(* Logix 5000 Rung export; software revision 16.04 *)

TYPE MNETCDATETIME :   // Stores the date and time value
STRUCT
   Year : DINT;   // Displays module current year
   Month : DINT;   // Displays Module current month
   Day : DINT;   // Displays Module current day
   Hour : DINT;   // Displays Module current hour
   Minute : DINT;   // Displays Module current minute
   Seconds : DINT;   // Displays Module current second
END_STRUCT
END_TYPE

TYPE MNETCETHERNETTYPE :   // Allows read/write Ethernet settings between the module and processor
STRUCT
   Read : BOOL;   // Enable Ethernet configuration transfer from module to processor
   Write : BOOL;   // Enable Ethernet configuration transfer from processor to module
   Config : MNETCETHERNET;   // Module ethernet configurations ip, netmask and gateway
END_STRUCT
END_TYPE

TYPE MNETCCLOCKTYPE :   // Allows read/write of clock value between the module and processor
STRUCT
   Read : BOOL;   // Reads current time from the module
   Write : BOOL;   // Writes current time from the module
   Config : MNETCDATETIME;   // Date and time configuration read or written between the module and processor
END_STRUCT
END_TYPE

TYPE MNETCETHERNET :   // Stores the MVI56E-MNETC IP settings
STRUCT
   IP : INT[4];   // Module IP address
   Netmask : INT[4];   // Net mask used by the Module
   Gateway : INT[4];   // Gateway used by the module
END_STRUCT
END_TYPE

ADD_ON_INSTRUCTION AOI56EMNETC_Optional   (* revision 1.0, vendor ProSoft Technology Inc. *)
// MVI56E-MNETC Optional Add-On Ethernet/Clock
// Revision note:
// v1.0 - Release.
VAR_IN_OUT
   MVI56MNETCEthernet : MNETCETHERNETTYPE; {required}   // MVI56E-MNET Rev2 Ethernet Settings
   MVI56MNETCClock : MNETCCLOCKTYPE; {required}   // MVI56E-MNET Rev2 Clock Settings
   ReadEthernetMSG : MESSAGE; {required}   // Read Ethernet Settings Message
   WriteEthernetMSG : MESSAGE; {required}   // Write Ethernet Settings Message
   ReadClockMSG : MESSAGE; {required}   // Read Clock Settings Message
   WriteClockMSG : MESSAGE; {required}   // Write Clock Settings Message
END_VAR

ROUTINE Logic   (* ladder *)
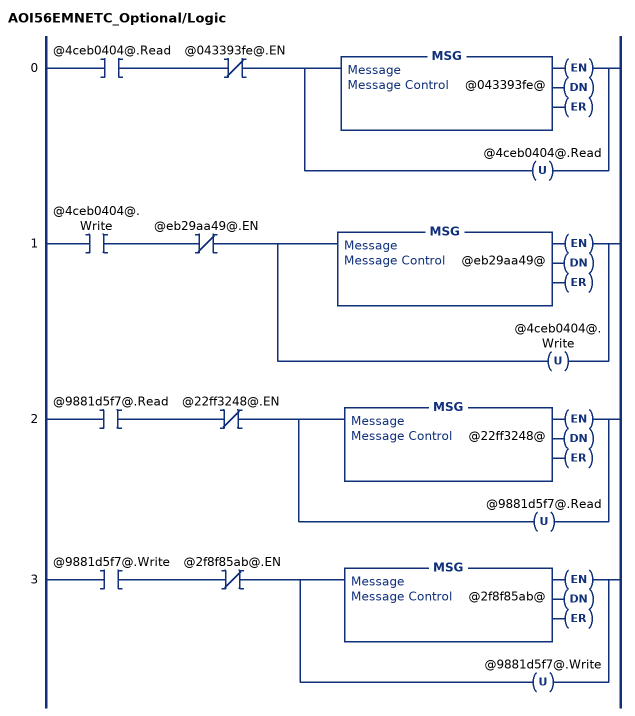
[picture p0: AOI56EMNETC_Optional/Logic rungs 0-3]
   0: XIC(@4ceb0404@.Read)XIO(@043393fe@.EN)[MSG(@043393fe@) ,OTU(@4ceb0404@.Read) ];
   1: XIC(@4ceb0404@.Write)XIO(@eb29aa49@.EN)[MSG(@eb29aa49@) ,OTU(@4ceb0404@.Write) ];
   2: XIC(@9881d5f7@.Read)XIO(@22ff3248@.EN)[MSG(@22ff3248@) ,OTU(@9881d5f7@.Read) ];
   3: XIC(@9881d5f7@.Write)XIO(@2f8f85ab@.EN)[MSG(@2f8f85ab@) ,OTU(@9881d5f7@.Write) ];
END_ROUTINE
END_ADD_ON_INSTRUCTION

VAR_GLOBAL   (* controller tags *)
   MVI56EMNETCETHERNET : MNETCETHERNETTYPE;
   READETHERNETMSG : MESSAGE;
        MessageParameters(MessageType := CIP Generic, ConnectedFlag := 2, ConnectionPath := MNETC, ServiceCode := 16#000e, ObjectType := 16#0004, TargetObject := 8, DestinationTag := MVI56EMNETCETHERNET.Config)
   WRITECLOCKMSG : MESSAGE;
        MessageParameters(MessageType := CIP Generic, RequestedLength := 24, ConnectedFlag := 2, ConnectionPath := MNETC, ServiceCode := 16#0010, ObjectType := 16#0004, TargetObject := 8, AttributeNumber := 16#0020, LocalElement := MVI56EMNETCCLOCK.Config)
   WRITEETHERNETMSG : MESSAGE;
        MessageParameters(MessageType := CIP Generic, RequestedLength := 24, ConnectedFlag := 2, ConnectionPath := MNETC, ServiceCode := 16#0010, ObjectType := 16#0004, TargetObject := 8, LocalElement := MVI56EMNETCETHERNET.Config)
   AOI56EMNETC_OPTIONAL : AOI56EMNETC_Optional;
   MVI56EMNETCCLOCK : MNETCCLOCKTYPE;
   READCLOCKMSG : MESSAGE;
        MessageParameters(MessageType := CIP Generic, ConnectedFlag := 2, ConnectionPath := MNETC, ServiceCode := 16#000e, ObjectType := 16#0004, TargetObject := 8, AttributeNumber := 16#0020, DestinationTag := MVI56EMNETCCLOCK.Config)
END_VAR

PROGRAM MainProgram

ROUTINE MainRoutine   (* ladder *)
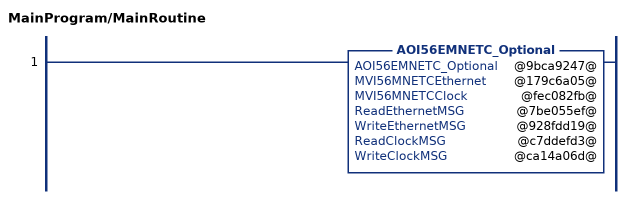
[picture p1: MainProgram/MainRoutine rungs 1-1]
   1: AOI56EMNETC_Optional(@9bca9247@,@179c6a05@,@fec082fb@,@7be055ef@,@928fdd19@,@c7ddefd3@,@ca14a06d@);
END_ROUTINE
END_PROGRAM
